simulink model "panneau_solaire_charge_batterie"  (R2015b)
settings: Solver=VariableStepAuto  StartTime=0.0  StopTime=83000  RelTol=1e-3
libraries: elec_lib x74, fl_lib x4, nesl_utility x3, powerlib_meascontrol x1

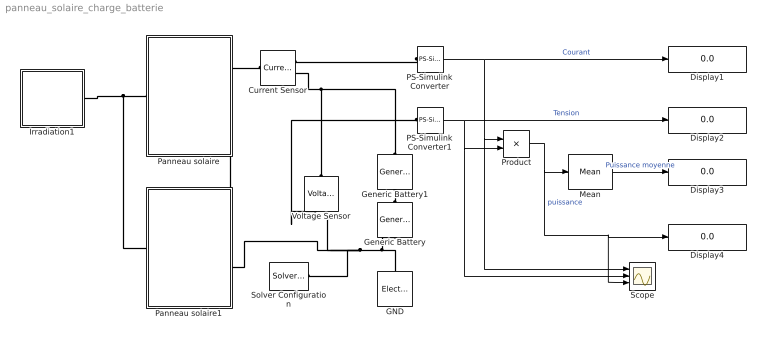
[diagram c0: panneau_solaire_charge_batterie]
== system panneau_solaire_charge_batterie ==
  Current Sensor : fl_lib/Electrical/Electrical Sensors/Current Sensor
  Display{1..4} (4 alike) : Display
  GND : fl_lib/Electrical/Electrical Elements/Electrical Reference
  Generic Battery : elec_lib/Sources/Generic Battery  Vnom=14.5 V  R1=0.0058 Ohm  prm_AH=2  AH=83 hr*A  AH0=1 hr*A  V1=11.5 V  AH1=15 hr*A  prm_R2=1  R2=2e+3 Ohm
  Generic Battery1 : elec_lib/Sources/Generic Battery  Vnom=14.5 V  R1=0.0058 Ohm  prm_AH=2  AH=83 hr*A  AH0=1 hr*A  V1=11.5 V  AH1=15 hr*A  prm_R2=1  R2=2e+3 Ohm
  Irradiation1 : Subsystem
  Mean : powerlib_meascontrol/Measurements/Mean  Freq=1/83000  Vinit=0  Ts=0
  PS-Simulink Converter : nesl_utility/PS-Simulink Converter  PhysicalDomain=network_engine_domain  SubClassName=ps_output  LeftPortType=input  RightPortType=output  PseudoPeriodic=off  Frequencies=[]  Unit=1  AffineConversion=off
  PS-Simulink Converter1 : nesl_utility/PS-Simulink Converter  PhysicalDomain=network_engine_domain  SubClassName=ps_output  LeftPortType=input  RightPortType=output  PseudoPeriodic=off  Frequencies=[]  Unit=1  AffineConversion=off
  Panneau solaire : Subsystem
  Panneau solaire1 : Subsystem
  Product : Product
  Scope : Scope  NumInputPorts=3
  Solver Configuration : nesl_utility/Solver Configuration  PhysicalDomain=network_engine_domain  SubClassName=solver  LeftPortType=input  RightPortType=generic  Accelerate=off  Tones=[]  Harmonics=[]  SimulateNoise=off  Profile=off  UseLocalSampling=off  EnableSwitchedLinearOptims=on  FrequencyDomain=off  UseCCode=off  RelTol=0.001  AbsTol=1e-06  MinStep=1e-09  ToWorkspace=off  RevertToSquareIcSolve=off  NumHomotopyIterations=100  PhasorMode=off  PhasorModeNumHarmonics=1  DoDC=off  ResidualTolerance=1e-9  UseLocalSolver=off  LocalSolverChoice=NE_BACKWARD_EULER_ADVANCER  LocalSolverSampleTime=.001  DoFixedCost=off  MaxNonlinIter=3  MaxModeIter=2  LinearAlgebra=Sparse  DelaysMemoryBudget=1024  AutomaticFiltering=on  FilteringTimeConstant=0.001
  Voltage Sensor : fl_lib/Electrical/Electrical Sensors/Voltage Sensor
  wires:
  PS-Simulink Converter/1 -> Display1/1, Product/1, Scope/1  "Courant"
  PS-Simulink Converter1/1 -> Display2/1, Product/2, Scope/2  "Tension"
  Product/1 -> Scope/3, Display4/1, Mean/1  "puissance"
  Mean/1 -> Display3/1  "Puissance moyenne"
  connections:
  Generic Battery1/LConn1 -- Current Sensor/RConn2 -- Voltage Sensor/LConn1
  Solver Configuration/RConn1 -- GND/LConn1 -- Generic Battery/RConn1 -- Voltage Sensor/RConn2 -- Panneau solaire1/RConn2
  Panneau solaire/LConn1 -- Irradiation1/RConn1 -- Panneau solaire1/LConn1
  PS-Simulink Converter/LConn1 -- Current Sensor/RConn1
  PS-Simulink Converter1/LConn1 -- Voltage Sensor/RConn1
  Panneau solaire/RConn2 -- Panneau solaire1/RConn1
  Panneau solaire/RConn1 -- Current Sensor/LConn1
  Generic Battery/LConn1 -- Generic Battery1/RConn1

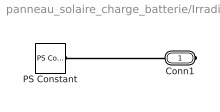
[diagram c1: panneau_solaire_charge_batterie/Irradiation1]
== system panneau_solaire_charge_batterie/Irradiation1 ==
  PS Constant : fl_lib/Physical Signals/Sources/PS Constant  constant=E
  Conn1 : PMIOPort  Port=1  Side=Right
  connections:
  Conn1/RConn1 -- PS Constant/RConn1

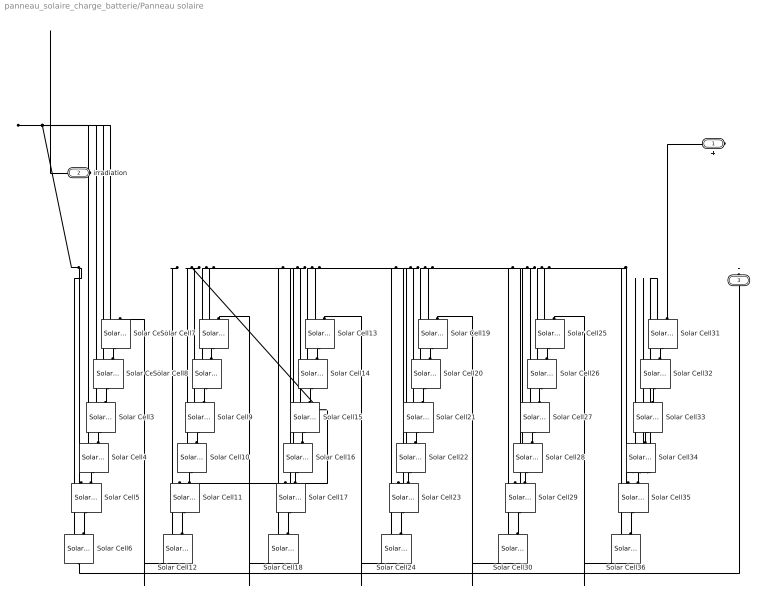
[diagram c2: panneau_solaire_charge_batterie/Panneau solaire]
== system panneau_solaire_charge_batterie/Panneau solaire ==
  Solar Cell{1..4,6..36} (35 alike) : elec_lib/Sources/Solar Cell  prm=1  Isc=Isc A  Voc=0.6 V  Is=1e-6 A  Is2=0 A  Iph=7.34 A  Ir0=1000 W/m^2  ec=1.5  N2=2  Rs=0 Ohm  Rp=Inf Ohm  N_series=1  TIPH1=0 1/K  EG=1.11 eV  TXIS1=3  TXIS2=3  TRS1=0  TRP1=0  Tmeas=25 C  TFIXED=Tcell C  thermal_mass=100 J/K  initial_temperature=25 C
  Solar Cell5 : elec_lib/Sources/Solar Cell  prm=1  Isc=Isc A  Voc=0.6 V  Is=1e-6 A  Is2=0 A  Iph=7.34 A  Ir0=1000 W/m^2  ec=1.5  N2=2  Rs=0 Ohm  Rp=Inf Ohm  N_series=1  TIPH1=0 1/K  EG=1.11 eV  TXIS1=3  TXIS2=3  TRS1=0  TRP1=0  Tmeas=25 C  TFIXED=25 C  thermal_mass=100 J/K  initial_temperature=25 C
  + : PMIOPort  Port=1  Side=Right
  irradiation : PMIOPort  Port=2  Side=Left
  - : PMIOPort  Port=3  Side=Right
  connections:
  Solar Cell6/RConn1 -- -/RConn1
  Solar Cell31/LConn2 -- +/RConn1
  Solar Cell35/LConn1 -- Solar Cell25/LConn1 -- Solar Cell30/LConn1 -- Solar Cell19/LConn1 -- Solar Cell24/LConn1 -- Solar Cell13/LConn1 -- Solar Cell18/LConn1 -- Solar Cell7/LConn1 -- Solar Cell12/LConn1 -- irradiation/RConn1 -- Solar Cell1/LConn1 -- Solar Cell2/LConn1 -- Solar Cell3/LConn1 -- Solar Cell6/LConn1 -- Solar Cell5/LConn1 -- Solar Cell4/LConn1 -- Solar Cell11/LConn1 -- Solar Cell10/LConn1 -- Solar Cell9/LConn1 -- Solar Cell8/LConn1 -- Solar Cell17/LConn1 -- Solar Cell16/LConn1 -- Solar Cell15/LConn1 -- Solar Cell14/LConn1 -- Solar Cell23/LConn1 -- Solar Cell22/LConn1 -- Solar Cell21/LConn1 -- Solar Cell20/LConn1 -- Solar Cell29/LConn1 -- Solar Cell28/LConn1 -- Solar Cell27/LConn1 -- Solar Cell26/LConn1 -- Solar Cell36/LConn1 -- Solar Cell31/LConn1 -- Solar Cell32/LConn1 -- Solar Cell33/LConn1 -- Solar Cell34/LConn1
  Solar Cell4/LConn2 -- Solar Cell3/RConn1
  Solar Cell2/LConn2 -- Solar Cell1/RConn1
  Solar Cell3/LConn2 -- Solar Cell2/RConn1
  Solar Cell5/LConn2 -- Solar Cell4/RConn1
  Solar Cell1/LConn2 -- Solar Cell12/RConn1
  Solar Cell6/LConn2 -- Solar Cell5/RConn1
  Solar Cell12/LConn2 -- Solar Cell11/RConn1
  Solar Cell9/LConn2 -- Solar Cell8/RConn1
  Solar Cell10/LConn2 -- Solar Cell9/RConn1
  Solar Cell8/LConn2 -- Solar Cell7/RConn1
  Solar Cell11/LConn2 -- Solar Cell10/RConn1
  Solar Cell7/LConn2 -- Solar Cell18/RConn1
  Solar Cell18/LConn2 -- Solar Cell17/RConn1
  Solar Cell15/LConn2 -- Solar Cell14/RConn1
  Solar Cell16/LConn2 -- Solar Cell15/RConn1
  Solar Cell14/LConn2 -- Solar Cell13/RConn1
  Solar Cell17/LConn2 -- Solar Cell16/RConn1
  Solar Cell13/LConn2 -- Solar Cell24/RConn1
  Solar Cell20/LConn2 -- Solar Cell19/RConn1
  Solar Cell23/LConn2 -- Solar Cell22/RConn1
  Solar Cell24/LConn2 -- Solar Cell23/RConn1
  Solar Cell19/LConn2 -- Solar Cell30/RConn1
  Solar Cell21/LConn2 -- Solar Cell20/RConn1
  Solar Cell22/LConn2 -- Solar Cell21/RConn1
  Solar Cell28/LConn2 -- Solar Cell27/RConn1
  Solar Cell30/LConn2 -- Solar Cell29/RConn1
  Solar Cell25/LConn2 -- Solar Cell36/RConn1
  Solar Cell27/LConn2 -- Solar Cell26/RConn1
  Solar Cell26/LConn2 -- Solar Cell25/RConn1
  Solar Cell29/LConn2 -- Solar Cell28/RConn1
  Solar Cell34/LConn2 -- Solar Cell33/RConn1
  Solar Cell36/LConn2 -- Solar Cell35/RConn1
  Solar Cell35/LConn2 -- Solar Cell34/RConn1
  Solar Cell32/LConn2 -- Solar Cell31/RConn1
  Solar Cell33/LConn2 -- Solar Cell32/RConn1

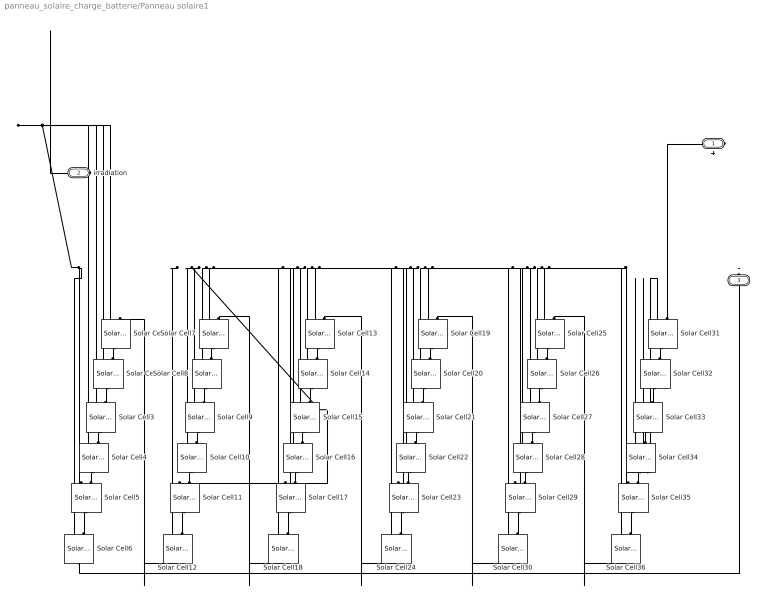
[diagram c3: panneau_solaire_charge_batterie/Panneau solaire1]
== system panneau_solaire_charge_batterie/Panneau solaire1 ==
  Solar Cell{1..4,6..36} (35 alike) : elec_lib/Sources/Solar Cell  prm=1  Isc=Isc A  Voc=0.6 V  Is=1e-6 A  Is2=0 A  Iph=7.34 A  Ir0=1000 W/m^2  ec=1.5  N2=2  Rs=0 Ohm  Rp=Inf Ohm  N_series=1  TIPH1=0 1/K  EG=1.11 eV  TXIS1=3  TXIS2=3  TRS1=0  TRP1=0  Tmeas=25 C  TFIXED=Tcell C  thermal_mass=100 J/K  initial_temperature=25 C
  Solar Cell5 : elec_lib/Sources/Solar Cell  prm=1  Isc=Isc A  Voc=0.6 V  Is=1e-6 A  Is2=0 A  Iph=7.34 A  Ir0=1000 W/m^2  ec=1.5  N2=2  Rs=0 Ohm  Rp=Inf Ohm  N_series=1  TIPH1=0 1/K  EG=1.11 eV  TXIS1=3  TXIS2=3  TRS1=0  TRP1=0  Tmeas=25 C  TFIXED=25 C  thermal_mass=100 J/K  initial_temperature=25 C
  + : PMIOPort  Port=1  Side=Right
  irradiation : PMIOPort  Port=2  Side=Left
  - : PMIOPort  Port=3  Side=Right
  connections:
  Solar Cell6/RConn1 -- -/RConn1
  Solar Cell31/LConn2 -- +/RConn1
  Solar Cell35/LConn1 -- Solar Cell25/LConn1 -- Solar Cell30/LConn1 -- Solar Cell19/LConn1 -- Solar Cell24/LConn1 -- Solar Cell13/LConn1 -- Solar Cell18/LConn1 -- Solar Cell7/LConn1 -- Solar Cell12/LConn1 -- irradiation/RConn1 -- Solar Cell1/LConn1 -- Solar Cell2/LConn1 -- Solar Cell3/LConn1 -- Solar Cell6/LConn1 -- Solar Cell5/LConn1 -- Solar Cell4/LConn1 -- Solar Cell11/LConn1 -- Solar Cell10/LConn1 -- Solar Cell9/LConn1 -- Solar Cell8/LConn1 -- Solar Cell17/LConn1 -- Solar Cell16/LConn1 -- Solar Cell15/LConn1 -- Solar Cell14/LConn1 -- Solar Cell23/LConn1 -- Solar Cell22/LConn1 -- Solar Cell21/LConn1 -- Solar Cell20/LConn1 -- Solar Cell29/LConn1 -- Solar Cell28/LConn1 -- Solar Cell27/LConn1 -- Solar Cell26/LConn1 -- Solar Cell36/LConn1 -- Solar Cell31/LConn1 -- Solar Cell32/LConn1 -- Solar Cell33/LConn1 -- Solar Cell34/LConn1
  Solar Cell4/LConn2 -- Solar Cell3/RConn1
  Solar Cell2/LConn2 -- Solar Cell1/RConn1
  Solar Cell3/LConn2 -- Solar Cell2/RConn1
  Solar Cell5/LConn2 -- Solar Cell4/RConn1
  Solar Cell1/LConn2 -- Solar Cell12/RConn1
  Solar Cell6/LConn2 -- Solar Cell5/RConn1
  Solar Cell12/LConn2 -- Solar Cell11/RConn1
  Solar Cell9/LConn2 -- Solar Cell8/RConn1
  Solar Cell10/LConn2 -- Solar Cell9/RConn1
  Solar Cell8/LConn2 -- Solar Cell7/RConn1
  Solar Cell11/LConn2 -- Solar Cell10/RConn1
  Solar Cell7/LConn2 -- Solar Cell18/RConn1
  Solar Cell18/LConn2 -- Solar Cell17/RConn1
  Solar Cell15/LConn2 -- Solar Cell14/RConn1
  Solar Cell16/LConn2 -- Solar Cell15/RConn1
  Solar Cell14/LConn2 -- Solar Cell13/RConn1
  Solar Cell17/LConn2 -- Solar Cell16/RConn1
  Solar Cell13/LConn2 -- Solar Cell24/RConn1
  Solar Cell20/LConn2 -- Solar Cell19/RConn1
  Solar Cell23/LConn2 -- Solar Cell22/RConn1
  Solar Cell24/LConn2 -- Solar Cell23/RConn1
  Solar Cell19/LConn2 -- Solar Cell30/RConn1
  Solar Cell21/LConn2 -- Solar Cell20/RConn1
  Solar Cell22/LConn2 -- Solar Cell21/RConn1
  Solar Cell28/LConn2 -- Solar Cell27/RConn1
  Solar Cell30/LConn2 -- Solar Cell29/RConn1
  Solar Cell25/LConn2 -- Solar Cell36/RConn1
  Solar Cell27/LConn2 -- Solar Cell26/RConn1
  Solar Cell26/LConn2 -- Solar Cell25/RConn1
  Solar Cell29/LConn2 -- Solar Cell28/RConn1
  Solar Cell34/LConn2 -- Solar Cell33/RConn1
  Solar Cell36/LConn2 -- Solar Cell35/RConn1
  Solar Cell35/LConn2 -- Solar Cell34/RConn1
  Solar Cell32/LConn2 -- Solar Cell31/RConn1
  Solar Cell33/LConn2 -- Solar Cell32/RConn1
